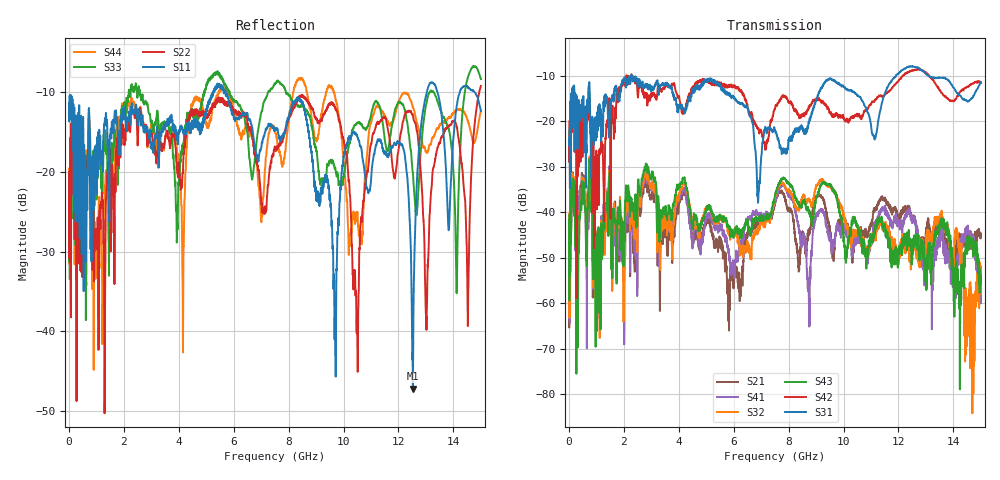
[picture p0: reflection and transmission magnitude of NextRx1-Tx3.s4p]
! FILE: N:\QM 2007\Prüfprotokolle\Highspeed\Konfektionierte Ltg\L45593-D106\D30\8216\0002\Next  Platine 2\NextRx1-Tx3.s4p
# MHz S DB R 50.00
! FREQ  S11  S12  S13  S14
!  S21  S22  S23  S24
!  S31  S32  S33  S34
!  S41  S42  S43  S44
!  DB  ANG  DB  ANG  DB  ANG  DB  ANG
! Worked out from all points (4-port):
!   2999 points, 10 MHz to 15 GHz, reference 50 ohm
!   strongest paths, dB at 10 MHz, 3.755 GHz, 7.505 GHz, 11.26 GHz, 15 GHz:
!     S31: -23.9, -12.7, -22.1, -20.2, -11.4
!     S42: -24.9, -11.7, -17.4, -14.7, -11.7
!     S43: -41.8, -41.6, -36.3, -42.0, -55.1
!     S32: -43.3, -47.8, -36.4, -43.2, -57.9
!     S41: -51.7, -42.5, -37.5, -41.3, -58.1
!     S21: -52.6, -48.0, -38.2, -38.3, -45.2
!   lowest |S11| = -47.2 dB at 12.53 GHz (marker M1), VSWR 1.01, Z = 49.6 + j0.202 ohm
!   |S11| at or under -10 dB: start of sweep to 5.257 GHz; 5.703 GHz to 13.03 GHz (7.331 GHz wide, 78.3 % of centre); 13.41 GHz to 14.23 GHz (817.5 MHz wide, 5.92 % of centre)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
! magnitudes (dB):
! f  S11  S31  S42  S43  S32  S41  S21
! 10 MHz  -11.4  -23.9  -24.9  -41.8  -43.3  -51.7  -52.6
! 6.905 GHz  -18.7  -35.5  -21.5  -41.3  -43.2  -40.2  -43.4
! 9.59 GHz  -28.1  -11.1  -19.0  -34.9  -35.4  -47.4  -48.3
! 10.49 GHz  -15.4  -14.3  -18.4  -42.9  -44.4  -45.2  -44.9
! 12.53 GHz  -47.2  -8.0  -8.9  -47.3  -47.0  -41.5  -41.8
! 13.03 GHz  -10.2  -9.8  -9.5  -56.6  -45.4  -52.5  -43.7
! 15 GHz  -12.4  -11.4  -11.7  -55.1  -57.9  -58.1  -45.2
